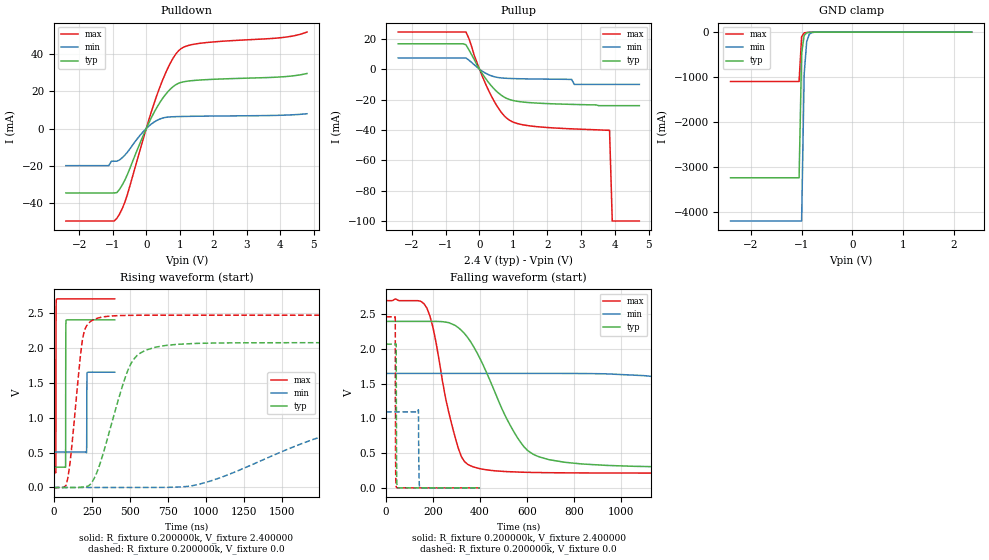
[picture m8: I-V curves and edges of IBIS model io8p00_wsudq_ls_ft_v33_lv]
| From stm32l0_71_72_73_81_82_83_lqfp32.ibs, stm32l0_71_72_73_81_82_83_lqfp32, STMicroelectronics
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|   Model io8p00_wsudq_ls_ft_v33_lv
[Model]  io8p00_wsudq_ls_ft_v33_lv
Model_type I/O
Polarity   Non-Inverting
Enable   Active-Low
Vinl =   0.720000V
Vinh =   1.680000V
Vmeas =  1.200000V
Cref =   50.000000pF
Rref =   100.000000M
Vref =   0.0V
C_comp   2.582000pF   2.574200pF   2.601000pF
[Temperature Range]   25.000000   0.105000k   -40.000000
[Pullup Reference]   2.400000V   1.650000V   2.700000V
[Pulldown Reference]   0.0V   0.0V   0.0V
[POWER Clamp Reference]   2.400000V   1.650000V   2.700000V
[GND Clamp Reference]   0.0V   0.0V   0.0V
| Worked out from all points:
|   slope of the pulldown table from 0 to 0.36 V, typ, clamps not added: 28.5 ohm
|   slope of the pullup table from 0 to 0.36 V, typ, clamps not added: 32.2 ohm
|   GND clamp passes 1 mA (typ) near -0.65 V on its own axis
|   rising waveform, R_fixture 0.200000k, V_fixture 2.400000: 20-80 % time 676ps typ, 829ps min, 649ps max; typ from 0.291 V to 2.4 V
|   rising waveform, R_fixture 0.200000k, V_fixture 0.0: 20-80 % time 169ns typ, 817ns min, 66.4ns max; typ from 0 V to 2.07 V
|   falling waveform, R_fixture 0.200000k, V_fixture 2.400000: 20-80 % time 179ns typ, 726ns min, 89.5ns max; typ from 2.4 V to 0.291 V
|   falling waveform, R_fixture 0.200000k, V_fixture 0.0: 20-80 % time 1.2ns typ, 1.73ns min, 981ps max; typ from 2.07 V to 0 V
[Pulldown]
|Voltage   I(typ)   I(min)   I(max)
-2.4V     -34.7mA    -20mA      -49.82mA
-1.12V    -34.7mA    -20mA      -49.82mA
-1.04V    -34.7mA    -17.6mA    -49.82mA
-880mV    -34.55mA   -17.6mA    -48.46mA
-560mV    -24.65mA   -12.68mA   -35.33mA
0V        0A         0A         142fA
400mV     13.84mA    5.066mA    22.03mA
720mV     21.24mA    6.254mA    35.26mA
1.04V     24.82mA    6.464mA    43.03mA
1.6V      26.11mA    6.627mA    45.88mA
4V        27.76mA    7.125mA    48.87mA
4.8V      29.63mA    7.94mA     51.96mA
[Pullup]
|Voltage   I(typ)   I(min)   I(max)
-2.4V     16.77mA    7.419mA    24.51mA
-400mV    16.1mA     7.419mA    24.51mA
0V        -580fA     6.14pA     0A
320mV     -10.16mA   -4.078mA   -16.34mA
640mV     -17.08mA   -5.718mA   -28.28mA
960mV     -20.45mA   -6.128mA   -34.49mA
1.76V     -22.39mA   -6.47mA    -37.97mA
2.72V     -23.16mA   -6.7mA     -39.27mA
2.8V      -23.2mA    -10mA      -39.35mA
3.84V     -24mA      -10mA      -40.2mA
3.92V     -24mA      -10mA      -100mA
4.72V     -24mA      -10mA      -100mA
[GND_clamp]
|Voltage   I(typ)   I(min)   I(max)
-2.4V     -3.237A    -4.198A    -1.1A
-1.05V    -3.237A    -4.198A    -1.1A
-1V       -475.9mA   -4.198A    -104.3mA
-950mV    -76.36mA   -935.5mA   -18.56mA
-900mV    -16.77mA   -213mA     -9.293mA
-850mV    -6.713mA   -51.08mA   -6.724mA
-800mV    -4.108mA   -13.94mA   -4.924mA
-650mV    -1.048mA   -1.2mA     -1.149mA
2.35V     0A         0A         0A
[POWER_clamp]
|Voltage   I(typ)   I(min)   I(max)
-2.4V     0A         0A         0A
0V        0A         0A         0A
[Ramp]
| variable   typ   min   max
dV/dt_r  0.65070/0.30199u   0.18995/0.81412u   1.03800/0.14355u
dV/dt_f  0.75690/0.32131u   0.19674/0.84507u   1.13815/0.15964u
R_load = 50.000000
[Rising Waveform]
R_fixture= 0.200000k
V_fixture= 2.400000
V_fixture_min= 1.650000
V_fixture_max= 2.700000
|time   V(typ)   V(min)   V(max)
0s        290.7mV    507.1mV    212.9mV
13.21ns   290.7mV    507.1mV    211.4mV
14.41ns   290.7mV    507.1mV    2.259V
16.82ns   290.7mV    507.1mV    2.691V
76.88ns   288.9mV    507.1mV    2.7V
78.48ns   2.092V     507.1mV    2.7V
80.88ns   2.392V     507.1mV    2.7V
215ns     2.4V       501.7mV    2.7V
219.4ns   2.4V       1.645V     2.7V
400ns     2.4V       1.65V      2.7V
[Rising Waveform]
R_fixture= 0.200000k
V_fixture= 0.0
V_fixture_min= 0.0
V_fixture_max= 0.0
|time   V(typ)   V(min)   V(max)
0s        1.941nV    12.05nV    1.476nV
93.43ns   -107.9uV   12.05nV    148mV
200.2ns   10.25mV    12.05nV    2.242V
280.3ns   201.2mV    -23.54uV   2.419V
373.7ns   869.2mV    -23.65uV   2.454V
547.2ns   1.889V     187.5uV    2.465V
934.3ns   2.062V     36.73mV    2.467V
1.989us   2.072V     869.4mV    2.467V
2.829us   2.072V     1.064V     2.467V
13.33us   2.072V     1.095V     2.467V
[Falling Waveform]
R_fixture= 0.200000k
V_fixture= 2.400000
V_fixture_min= 1.650000
V_fixture_max= 2.700000
|time   V(typ)   V(min)   V(max)
0s        2.4V       1.65V      2.7V
160.2ns   2.4V       1.65V      2.659V
320.3ns   2.274V     1.65V      452.1mV
507.2ns   1.042V     1.65V      235.4mV
613.9ns   512.1mV    1.65V      222.9mV
827.5ns   346.7mV    1.649V     215.2mV
1.348us   297mV      1.498V     213mV
2.202us   291mV      719.3mV    212.9mV
2.95us    290.7mV    552.4mV    212.9mV
13.33us   290.7mV    507.1mV    212.9mV
[Falling Waveform]
R_fixture= 0.200000k
V_fixture= 0.0
V_fixture_min= 0.0
V_fixture_max= 0.0
|time   V(typ)   V(min)   V(max)
0s        2.072V     1.095V     2.467V
38.44ns   2.072V     1.095V     2.467V
40.44ns   2.072V     1.095V     265.5mV
42.84ns   2.062V     1.095V     17.57mV
43.64ns   1.019V     1.095V     8.739mV
45.25ns   117.2mV    1.095V     2.426mV
48.85ns   6.179mV    1.095V     310.2uV
137.3ns   20.99uV    1.126V     134uV
144.1ns   21.24uV    5.499mV    135uV
400ns     1.941nV    12.05nV    1.476nV
